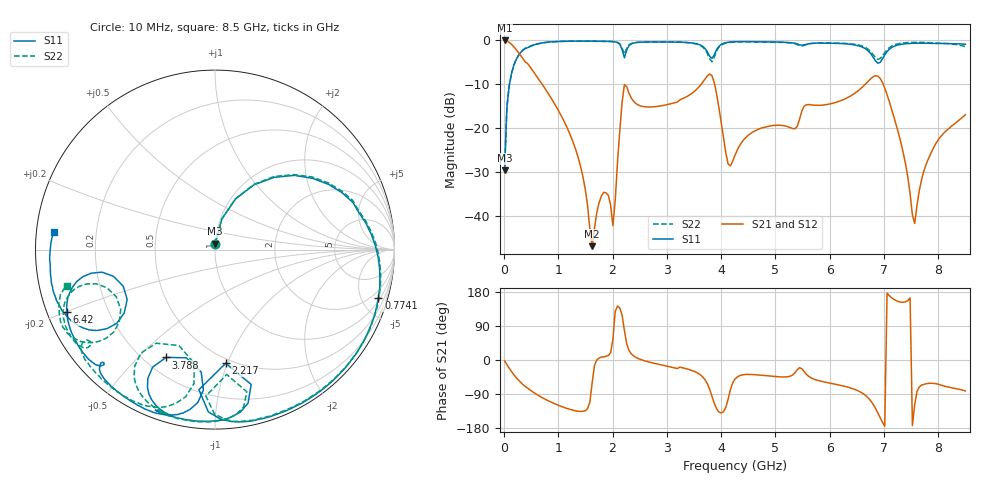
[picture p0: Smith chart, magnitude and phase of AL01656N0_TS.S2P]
!AVX CORPORATION
!PART NUMBER AL01656N0_TS
!DESCRIPTION: AIR CORE INDUCTOR, 56nH, 7 TURNS
!Agilent Technologies,E5071C,MY46102230,A.09.54
!Date: Mon Sep 03 16:37:34 2012
!Data & Calibration Information:
!Freq	S11:SOLT2(ON)	S21:SOLT2(ON)	S12:SOLT2(ON)	S22:SOLT2(ON)
# Hz S dB R 50
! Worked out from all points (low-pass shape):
!   201 points, 10 MHz to 8.5 GHz, reference 50 ohm
!   highest |S21| = -0.01 dB at 10 MHz (marker M1); lowest = -46.8 dB at 1.623 GHz (marker M2)
!   |S21| within 3 dB of the highest: start of sweep to 280.6 MHz
!   lowest |S11| = -29.5 dB at 10 MHz (marker M3), VSWR 1.07, Z = 50 + j3.35 ohm
!   |S11| at or under -10 dB: start of sweep to 99.62 MHz
!   |S22| runs from -29.4 to -0.2 dB; largest |S21 - S12| = 0.0068
!   S11 on the Smith chart (normalised r, x): 10 MHz: 1.00, +0.07; 774.1 MHz: 1.20, -6.64; 2.217 GHz: 0.46, -0.99; 3.788 GHz: 0.29, -0.61; 6.42 GHz: 0.06, -0.20; 8.5 GHz: 0.05, +0.05
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1e7  -29.50 87.6  -0.01 -2.3  -0.07 -2.3  -29.41 87.6
5.245e7  -15.15 77.4  -0.15 -12.2  -0.12 -12.2  -15.13 77.5
1.798e8  -5.66 50.6  -1.44 -38.6  -1.42 -38.7  -5.63 51.1
3.9205e8  -1.80 18.8  -4.92 -70.2  -4.90 -70.2  -1.78 19.6
7.741e8  -0.45 -16.6  -11.31 -104.8  -11.30 -104.9  -0.45 -15.6
1.4533e9  -0.15 -56.5  -31.01 -135.3  -31.03 -135.7  -0.19 -56.0
1.6231e9  -0.16 -64.3  -46.79 -60.5  -46.52 -59.9  -0.20 -63.9
1.83535e9  -0.19 -73.7  -34.54 8.0  -34.72 8.4  -0.22 -73.3
2.00515e9  -0.27 -82.2  -42.11 53.6  -42.08 52.7  -0.28 -81.2
2.2174e9  -3.93 -84.6  -10.02 77.8  -10.03 77.8  -3.11 -84.6
2.85415e9  -0.35 -100.7  -14.95 -11.5  -14.95 -11.6  -0.32 -100.1
3.78805e9  -3.61 -114.4  -7.64 -77.4  -7.64 -77.4  -4.21 -122.2
3.9154e9  -2.10 -94.7  -12.14 -128.5  -12.14 -128.5  -2.44 -98.9
4.12765e9  -0.42 -104.7  -28.09 -103.6  -28.09 -103.7  -0.52 -111.5
4.255e9  -0.30 -108.6  -26.11 -50.3  -26.11 -50.2  -0.39 -116.6
5.6983e9  -0.65 -137.3  -14.71 -49.9  -14.71 -49.9  -0.65 -145.0
6.41995e9  -0.95 -157.3  -12.38 -75.5  -12.37 -75.5  -0.81 -158.2
6.802e9  -3.85 -168.7  -8.26 -117.4  -8.26 -117.4  -3.26 -163.9
7.09915e9  -1.99 -145.5  -13.94 169.5  -13.95 169.4  -1.63 -141.8
7.5661e9  -0.65 -163.5  -41.62 -117.3  -41.92 -118.0  -0.43 -152.8
7.86325e9  -0.66 -171.3  -25.67 -61.4  -25.68 -61.6  -0.53 -157.1
8.5e9  -0.87 173.8  -16.89 -81.7  -16.91 -81.7  -1.41 -166.2
